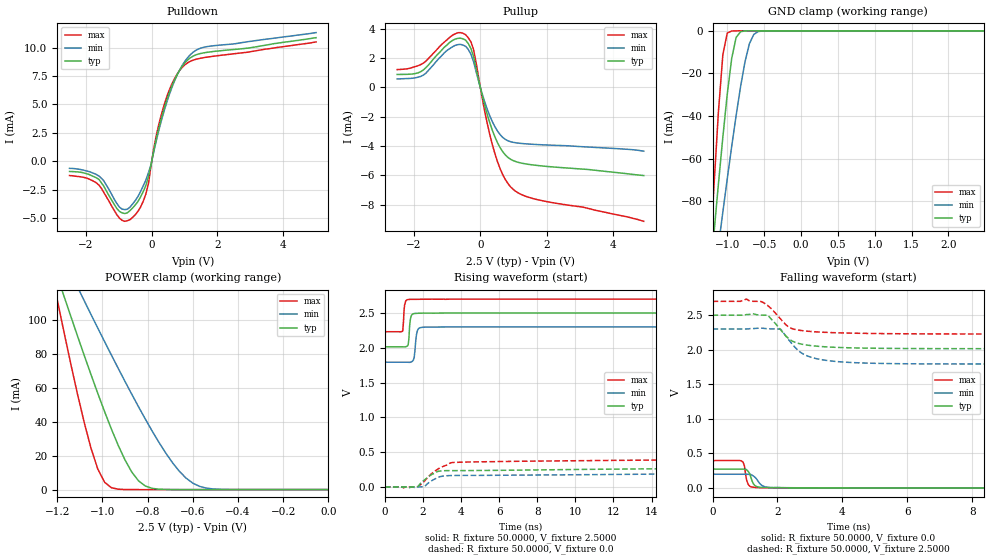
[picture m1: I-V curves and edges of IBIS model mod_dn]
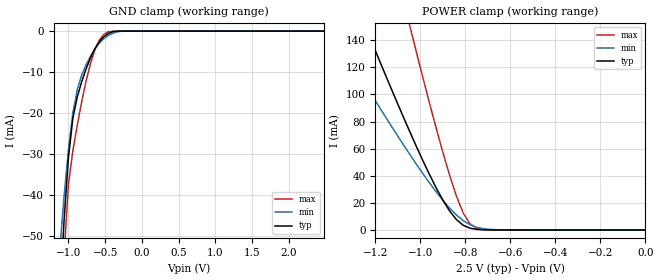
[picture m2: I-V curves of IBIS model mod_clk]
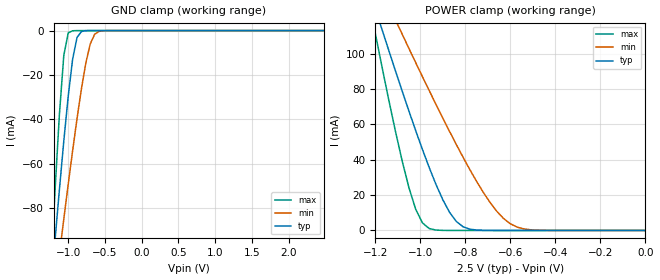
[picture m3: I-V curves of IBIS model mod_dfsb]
| IBIS (I/O, Buffer, Information, Specification) Model, officially
| electronic behavioral standard for Buffer structures of digital pins.
[IBIS ver]  4.0
[File name] rhf1401_2v5_rev3.ibs
[File Rev]  3.0
[Date]   26 Nov 2019
[Source]   CAD & Design Services (Catania) - STMicroelectronics
[Notes]
   (Note1) This IBIS model is the model of the product with package,
   SO48 ceramic package. This package model is defined between
   [Define Package Model] and [End Package Model] keywords;
   (Note2) This IBIS model is extracted with nominal 2.5V power supply
   (min:2.3V, typ:2.5V, max:2.7V);
   (Note3) This IBIS model has some Notes about the non-monotonicity
   of the I-V curves, but they are not indicative of problems
   inside the model;
[Copyright] (c) 2015 STMicroelectronics
|   Component RHF1401
[Component] RHF1401
[Manufacturer] STMicroelectronics
[Package]
| variable  typ   min   max
R_pkg   0.0   0.0   0.0
L_pkg   0.0H   0.0H   0.0H
C_pkg   0.0F   0.0F   0.0F
[Pin]   signal_name   model_name   R_pin   L_pin   C_pin
1   GNDBI   GND   NA   NA   NA
2   GBE1   GND   NA   NA   NA
3   VCBE1   POWER   NA   NA   NA
4   4   NC   NA   NA   NA
5   5   NC   NA   NA   NA
6   OR   mod_dn   NA   NA   NA
7   D13   mod_dn   NA   NA   NA
8   D12   mod_dn   NA   NA   NA
9   D11   mod_dn   NA   NA   NA
10   D10   mod_dn   NA   NA   NA
11   D9   mod_dn   NA   NA   NA
12   D8   mod_dn   NA   NA   NA
13   D7   mod_dn   NA   NA   NA
14   D6   mod_dn   NA   NA   NA
15   D5   mod_dn   NA   NA   NA
16   D4   mod_dn   NA   NA   NA
17   D3   mod_dn   NA   NA   NA
18   D2   mod_dn   NA   NA   NA
19   D1   mod_dn   NA   NA   NA
20   D0   mod_dn   NA   NA   NA
21   DR   mod_dn   NA   NA   NA
22   VCBE2   POWER   NA   NA   NA
23   GBE2   GND   NA   NA   NA
24   VCCBI   POWER   NA   NA   NA
25   DGND1   GND   NA   NA   NA
26   DGND2   GND   NA   NA   NA
27   CLK   mod_clk   NA   NA   NA
28   DGND3   GND   NA   NA   NA
29   DVCC1   POWER   NA   NA   NA
30   DVCC2   POWER   NA   NA   NA
31   AVCC1   POWER   NA   NA   NA
32   AVCC2   POWER   NA   NA   NA
33   AGND1   GND   NA   NA   NA
34   INCM   NC   NA   NA   NA
35   AGND2   GND   NA   NA   NA
36   VINB   NC   NA   NA   NA
37   AGND3   GND   NA   NA   NA
38   VIN   NC   NA   NA   NA
39   AGND4   GND   NA   NA   NA
40   VREFM   NC   NA   NA   NA
41   VREFP   NC   NA   NA   NA
42   IPOL   NC   NA   NA   NA
43   AGND5   GND   NA   NA   NA
44   AVCC   POWER   NA   NA   NA
45   AVCC   POWER   NA   NA   NA
46   DFSB   mod_dfsb   NA   NA   NA
47   OEB   mod_oeb   NA   NA   NA
48   REFMODE   NC   NA   NA   NA
[Package Model]   SO48
[Define Package Model]  SO48
[Manufacturer]  STMicroelectronics
[OEM]  STMicroelectronics
[Description]  48 ceramic package
[Number Of Pins]  48
[Pin Numbers]
|Pin Num   Terminal Name
1   | GNDBI
2   | GNDBE
3   | VCCBE
4   | NC
5   | NC
6   | OR
7   | D13
8   | D12
9   | D11
10   | D10
11   | D9
12   | D8
13   | D7
14   | D6
15   | D5
16   | D4
17   | D3
18   | D2
19   | D1
20   | D0
21   | DR
22   | VCCBE
23   | GNDBE
24   | VCCBI
25   | DGND
26   | DGND
27   | CLK
28   | DGND
29   | DVCC
30   | DVCC
31   | AVCC
32   | AVCC
33   | AGND
34   | INCM
35   | AGND
36   | VINB
37   | AGND
38   | VIN
39   | AGND
40   | VREFM
41   | VREFP
42   | IPOL
43   | AGND
44   | AVCC
45   | AVCC
46   | DFSB
47   | OEB
48   | REFMODE
[Model Data]
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[End Model Data]
[End Package Model]
| Models and submodels in the file (4): mod_dn (3-state), mod_clk (Input), mod_dfsb (Input), mod_oeb (Input)
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|   Model mod_dn
[Model]   mod_dn
Model_type 3-state
|Vinl   =   0.625V
|Vinh   =   1.875V
Vmeas  =   1.250V
Vref   =   2.500V
Cref   =   15pF
C_comp   0.508pF   0.485pF   0.532pF
[Temperature Range]  27.0000   0.1250k   -55.0000
[Voltage Range]   2.5000V   2.3000V   2.7000V
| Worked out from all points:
|   slope of the pulldown table from 0 to 0.375 V, typ, clamps not added: 81.1 ohm
|   slope of the pullup table from 0 to 0.375 V, typ, clamps not added: 125 ohm
|   GND clamp passes 1 mA (typ) near -0.83 V on its own axis
|   POWER clamp passes 1 mA (typ) near -0.79 V on its own axis
|   rising waveform, R_fixture 50.0000, V_fixture 2.5000: 20-80 % time 81.7ps typ, 115ps min, 70.6ps max; typ from 2.01 V to 2.5 V
|   rising waveform, R_fixture 50.0000, V_fixture 0.0: 20-80 % time 830ps typ, 850ps min, 1.24ns max; typ from 0 V to 0.268 V
|   falling waveform, R_fixture 50.0000, V_fixture 0.0: 20-80 % time 138ps typ, 210ps min, 93.8ps max; typ from 0.272 V to 0 V
|   falling waveform, R_fixture 50.0000, V_fixture 2.5000: 20-80 % time 632ps typ, 759ps min, 591ps max; typ from 2.5 V to 2.01 V
[Pulldown]
|Voltage   I(typ)   I(min)   I(max)
-2.5V     -901.1uA   -625.4uA   -1.257mA
-1.7V     -1.433mA   -1.142mA   -1.865mA
-1.46V    -2.182mA   -1.714mA   -2.733mA
-980mV    -4.422mA   -4.047mA   -5.01mA
-660mV    -4.348mA   -4.041mA   -5.14mA
-180mV    -2.148mA   -1.671mA   -2.909mA
140mV     1.978mA    1.811mA    2.279mA
300mV     3.846mA    3.634mA    4.182mA
620mV     6.673mA    6.533mA    6.849mA
940mV     8.417mA    8.495mA    8.305mA
1.58V     9.545mA    10.04mA    9.121mA
5V        10.88mA    11.33mA    10.51mA
[Pullup]
|Voltage   I(typ)   I(min)   I(max)
-2.5V     873.3uA    567.6uA    1.203mA
-1.8V     1.05mA     733.7uA    1.535mA
-920mV    3.06mA     2.632mA    3.402mA
-680mV    3.33mA     2.904mA    3.712mA
-440mV    3.209mA    2.787mA    3.579mA
-200mV    2.073mA    1.737mA    2.554mA
120mV     -1.115mA   -902.2uA   -1.48mA
440mV     -3.38mA    -2.688mA   -4.521mA
680mV     -4.405mA   -3.425mA   -5.973mA
920mV     -4.917mA   -3.717mA   -6.806mA
1.64V     -5.309mA   -3.895mA   -7.614mA
4.92V     -6.016mA   -4.356mA   -9.134mA
[GND_clamp]
|Voltage   I(typ)   I(min)   I(max)
-2.5V     -647mA     -491mA     -992.2mA
-1.24V    -118.3mA   -133.4mA   -110.2mA
-1.18V    -94.73mA   -117.1mA   -72.47mA
-1.12V    -71.78mA   -100.9mA   -37.89mA
-1.06V    -49.81mA   -84.98mA   -11.18mA
-1V       -29.61mA   -69.38mA   -1.046mA
-940mV    -12.92mA   -54.22mA   -82.43uA
-880mV    -3.113mA   -39.73mA   -10.57uA
-760mV    -46.21uA   -14.61mA   -27.16nA
-700mV    -4.665uA   -6.035mA   -1.125nA
-580mV    -45.36nA   -350.1uA   -8.653pA
2.48V     14.49pA    26.64nA    14.16pA
[POWER_clamp]
|Voltage   I(typ)   I(min)   I(max)
-2.49V    667.8mA    510.6mA    1.016A
-1.23V    137.7mA    152mA      131.4mA
-1.2V     125.7mA    143.7mA    111.8mA
-1.17V    113.8mA    135.5mA    92.69mA
-1.11V    90.3mA     119.1mA    56.09mA
-1.05V    67.48mA    102.9mA    24.14mA
-990mV    45.76mA    86.97mA    4.273mA
-900mV    17.47mA    63.64mA    48.56uA
-810mV    2.109mA    41.47mA    406nA
-660mV    7.7uA      10.86mA    158.5pA
-570mV    237.5nA    1.911mA    20.1pA
0V        14.61pA    65.38pA    15.5pA
[Ramp]
| variable   typ   min   max
dV/dt_r  0.1404/0.6726n   99.0778m/0.5948n   0.2116/0.9535n
dV/dt_f  0.2914/0.6727n   0.3042/0.8006n   0.2842/0.6044n
R_load = 50.0000
[Rising Waveform]
R_fixture= 50.0000
V_fixture= 2.5000
V_fixture_min= 2.3000
V_fixture_max= 2.7000
|time   V(typ)   V(min)   V(max)
0s        2.014V     1.793V     2.231V
940ps     2.014V     1.793V     2.241V
1.04ns    2.014V     1.793V     2.62V
1.18ns    2.025V     1.792V     2.692V
1.26ns    2.123V     1.791V     2.696V
1.34ns    2.413V     1.792V     2.697V
1.46ns    2.486V     1.811V     2.697V
1.7ns     2.496V     2.238V     2.697V
1.98ns    2.499V     2.295V     2.698V
20ns      2.5V       2.3V       2.7V
[Rising Waveform]
R_fixture= 50.0000
V_fixture= 0.0
V_fixture_min= 0.0
V_fixture_max= 0.0
|time   V(typ)   V(min)   V(max)
0s        5.501nV    388.2nV    1.872nV
980ps     337.4uV    -246.7nV   -14.34mV
1.3ns     -11.47mV   -195.8uV   35.92uV
1.74ns    5.72mV     -1.839mV   4.075mV
2.06ns    95.97mV    2.49mV     78.21mV
2.42ns    171.4mV    81.8mV     182.5mV
2.74ns    217.7mV    130.1mV    247.2mV
3.42ns    233.6mV    162.3mV    340.8mV
3.62ns    233.7mV    163.6mV    351.1mV
20ns      268.4mV    194mV      397.7mV
[Falling Waveform]
R_fixture= 50.0000
V_fixture= 0.0
V_fixture_min= 0.0
V_fixture_max= 0.0
|time   V(typ)   V(min)   V(max)
0s        271.9mV    197.2mV    395.7mV
880ps     271.8mV    197.2mV    393.1mV
980ps     269.8mV    197.1mV    322.1mV
1.04ns    265mV      197mV      138.6mV
1.1ns     237.2mV    195.8mV    50.48mV
1.26ns    57.74mV    171.2mV    9.441mV
1.42ns    10.76mV    85mV       3.374mV
1.66ns    5.913mV    11.96mV    1.424mV
2.34ns    905.1uV    2.055mV    485.5uV
20ns      12.03uV    18.26uV    7.171uV
[Falling Waveform]
R_fixture= 50.0000
V_fixture= 2.5000
V_fixture_min= 2.3000
V_fixture_max= 2.7000
|time   V(typ)   V(min)   V(max)
0s        2.5V       2.3V       2.7V
860ps     2.5V       2.3V       2.7V
1.04ns    2.509V     2.3V       2.733V
1.48ns    2.501V     2.314V     2.7V
1.7ns     2.5V       2.304V     2.64V
2.1ns     2.288V     2.297V     2.444V
2.42ns    2.135V     2.101V     2.311V
2.86ns    2.071V     1.923V     2.271V
4.18ns    2.028V     1.817V     2.241V
20ns      2.014V     1.793V     2.227V
|   Model mod_clk
[Model]   mod_clk
Model_type Input
Vinl   =   0.625V
Vinh   =   1.875V
C_comp   0.404pF   0.386pF   0.443pF
[Temperature Range]  27.0000   0.1250k   -55.0000
[Voltage Range]   2.5000V   2.3000V   2.7000V
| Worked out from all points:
|   GND clamp passes 1 mA (typ) near -0.49 V on its own axis
|   POWER clamp passes 1 mA (typ) near -0.77 V on its own axis
[GND_clamp]
|Voltage   I(typ)   I(min)   I(max)
-2.5V     -634.8mA   -434.7mA   -1.039A
-1.12V    -65.34mA   -53.42mA   -83.66mA
-1.06V    -46.02mA   -40.18mA   -54.43mA
-1V       -30.63mA   -28.68mA   -37.25mA
-940mV    -21.14mA   -19.87mA   -29.11mA
-880mV    -15.99mA   -14.2mA    -22.85mA
-760mV    -9.182mA   -8.171mA   -12.13mA
-640mV    -4.293mA   -4.347mA   -4.532mA
-580mV    -2.595mA   -2.942mA   -2.222mA
-460mV    -623.8uA   -1.096mA   -183.7uA
-220mV    -417.9nA   -8.331uA   -5.431nA
2.48V     474pA      21.04nA    14.16pA
[POWER_clamp]
|Voltage   I(typ)   I(min)   I(max)
-2.49V    674.6mA    459mA      1.167A
-1.41V    217.8mA    152.3mA    399.7mA
-1.38V    205.4mA    144mA      378.7mA
-1.23V    144.1mA    103.2mA    274.5mA
-1.05V    73.47mA    56.38mA    152.2mA
-1.02V    62.29mA    48.97mA    132.4mA
-930mV    31mA       28.09mA    75.02mA
-870mV    13.92mA    16.07mA    40.11mA
-810mV    3.466mA    6.921mA    12.52mA
-780mV    1.315mA    3.895mA    4.557mA
-690mV    45.39uA    399.6uA    52.87uA
0V        629.5pA    18.89nA    20.5pA
|   Model mod_dfsb
[Model]   mod_dfsb
Model_type Input
Vinl   =   0.625V
Vinh   =   1.875V
C_comp   0.508pF   0.485pF   0.532pF
[Temperature Range]  27.0000   0.1250k   -55.0000
[Voltage Range]   2.5000V   2.3000V   2.7000V
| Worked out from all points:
|   GND clamp passes 1 mA (typ) near -0.83 V on its own axis
|   POWER clamp passes 1 mA (typ) near -0.79 V on its own axis
[GND_clamp]
|Voltage   I(typ)   I(min)   I(max)
-2.5V     -647mA     -491mA     -992.2mA
-1.24V    -118.3mA   -133.4mA   -110.2mA
-1.18V    -94.73mA   -117.1mA   -72.47mA
-1.12V    -71.78mA   -100.9mA   -37.89mA
-1.06V    -49.81mA   -84.98mA   -11.18mA
-1V       -29.61mA   -69.38mA   -1.046mA
-940mV    -12.92mA   -54.22mA   -82.43uA
-880mV    -3.113mA   -39.73mA   -10.57uA
-760mV    -46.21uA   -14.61mA   -27.16nA
-700mV    -4.665uA   -6.035mA   -1.125nA
-580mV    -45.36nA   -350.1uA   -8.653pA
2.48V     14.49pA    26.64nA    14.16pA
[POWER_clamp]
|Voltage   I(typ)   I(min)   I(max)
-2.49V    667.8mA    510.6mA    1.016A
-1.23V    137.7mA    152mA      131.4mA
-1.2V     125.7mA    143.7mA    111.8mA
-1.17V    113.8mA    135.5mA    92.69mA
-1.11V    90.3mA     119.1mA    56.09mA
-1.05V    67.48mA    102.9mA    24.14mA
-990mV    45.76mA    86.97mA    4.273mA
-900mV    17.47mA    63.64mA    48.56uA
-810mV    2.109mA    41.47mA    406nA
-660mV    7.7uA      10.86mA    158.5pA
-570mV    237.5nA    1.911mA    20.1pA
0V        14.61pA    65.38pA    15.5pA
